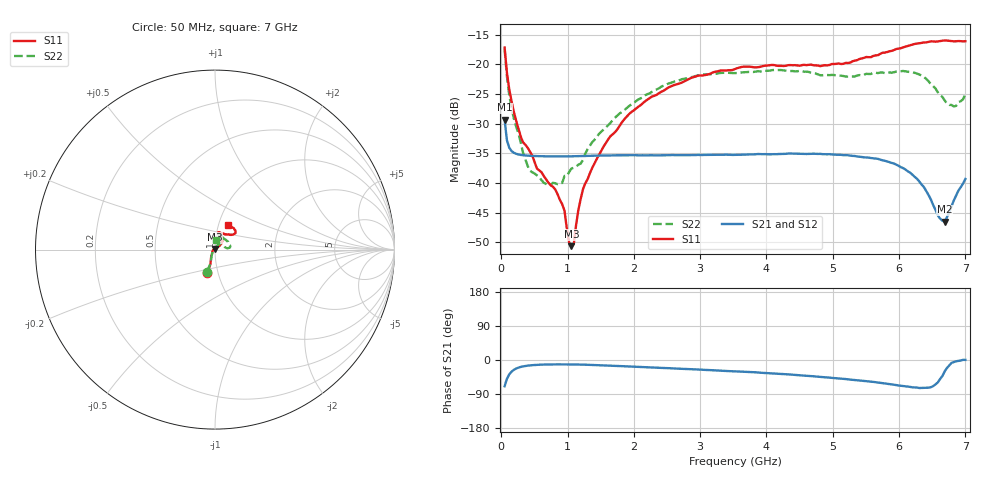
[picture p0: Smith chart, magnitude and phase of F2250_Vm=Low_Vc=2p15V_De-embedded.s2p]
! Integrated Device Technology
! Corporate Headquarters
! 6024 Silver Creek Valley Road
! San Jose, CA 95138  USA
! Phone:  1-408-284-8200
! Toll Free:  1-800-223-1366
! Webpage:  http://www.idt.com/
! Timing and RF Division
! 515 Groton Road, Suite 102
! Westford, MA 01886-6024
! Device:  F2250
! Description: Voltage Variable RF Attenuator
! Frequency:  50.0 -  6000.00 MHz
! Package:  3x3 mm Thin QFN Plastic Package: 16 pin
! Ports:  2 RF, 3 DC
!  Pin  1  = GND
!  Pin  2  = NC
!  Pin  3  = RF1  = Port 1
!  Pin  4  = NC
!  Pin  5  = GND
!  Pin  6  = GND
!  Pin  7  = GND
!  Pin  8  = GND
!  Pin  9  = NC
!  Pin 10  = RF2  = Port 2
!  Pin 11  = NC
!  Pin 12  = GND
!  Pin 13  = GND
!  Pin 14  = VCNTRL
!  Pin 15  = VDD
!  Pin 16  = VMODE
! Vcntrl:  2.150 Volts
! Vmode:  +0.000 Volts
! Vdd:  +3.30  Volts
! Current:  1.179 mA
! Data:  The device was measured on a the F2250 evaluation board which has
!  individual transmission lines to the RF pins.  Data was collected
!  using a calibrated network analyzer.  The evaluation board was
!  de-embedded using a TRL calibration technique.
!  The reference plane is the edge of the package pin.
! Misc:  SN 10
!  Action Tracker AT0258
! Date Measured:  2014-11-26
! Date:  2015-10-15  MJV
! Note:
!  Integrated Device Technology supplies this data as a sample of measured
!  data at the package pin for this product.  Your particular data for this
!  product may vary.
!  Data was taken at 25 degrees C.
!  Integrated Device Technology reserves the right to change this data at anytime.
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# GHz S dB R 50
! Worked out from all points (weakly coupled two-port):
!   201 points, 50 MHz to 7 GHz, reference 50 ohm
!   highest |S21| = -29.36 dB at 50 MHz (marker M1); lowest = -46.6 dB at 6.687 GHz (marker M2)
!   lowest |S11| = -50.7 dB at 1.058 GHz (marker M3), VSWR 1.01, Z = 49.8 + j0.247 ohm
!   |S11| at or under -10 dB: start of sweep to end of sweep
!   |S22| runs from -40.4 to -17.5 dB; largest |S21 - S12| = 5.8e-05
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0.05  -17.18 -108.6  -29.36 -69.2  -29.36 -69.2  -17.47 -110.1
0.08475  -21.44 -107.4  -32.82 -49.8  -32.82 -49.8  -22.03 -108.0
0.189  -28.00 -119.7  -34.92 -26.0  -34.92 -26.0  -29.14 -121.8
0.328  -33.16 -133.8  -35.35 -16.9  -35.34 -16.9  -34.90 -137.4
0.43225  -34.74 -144.6  -35.44 -14.2  -35.44 -14.2  -37.96 -162.7
0.71025  -39.96 -168.3  -35.53 -11.8  -35.53 -11.8  -40.39 150.5
0.91875  -43.61 158.1  -35.54 -11.6  -35.54 -11.6  -40.01 120.4
0.9535  -44.71 169.3  -35.54 -11.6  -35.54 -11.6  -38.83 119.3
1.023  -50.03 144.2  -35.53 -11.7  -35.53 -11.7  -38.18 101.0
1.05775  -50.68 122.1  -35.52 -11.7  -35.53 -11.7  -37.59 96.2
1.0925  -50.38 90.8  -35.51 -11.8  -35.51 -11.8  -37.45 91.3
1.162  -44.59 57.0  -35.50 -12.0  -35.50 -12.0  -36.94 79.9
1.2315  -41.10 44.2  -35.47 -12.2  -35.47 -12.2  -36.15 71.0
1.6485  -32.11 41.9  -35.38 -14.8  -35.38 -14.8  -29.85 57.1
2.37825  -24.87 47.3  -35.35 -20.5  -35.34 -20.5  -24.06 53.1
3.525  -20.80 72.5  -35.28 -29.9  -35.28 -29.9  -21.50 72.9
4.7065  -20.17 72.4  -35.09 -42.9  -35.09 -42.9  -21.52 71.2
5.85325  -17.82 40.5  -36.51 -63.5  -36.51 -63.6  -21.38 21.0
6.33975  -16.40 41.0  -40.29 -73.7  -40.30 -73.8  -21.89 6.9
6.68725  -15.99 48.8  -46.56 -30.3  -46.53 -29.9  -26.10 26.9
6.861  -16.12 55.1  -42.13 -3.4  -42.10 -3.3  -27.01 58.1
7  -16.12 63.3  -39.34 0.3  -39.30 0.2  -25.01 84.5
